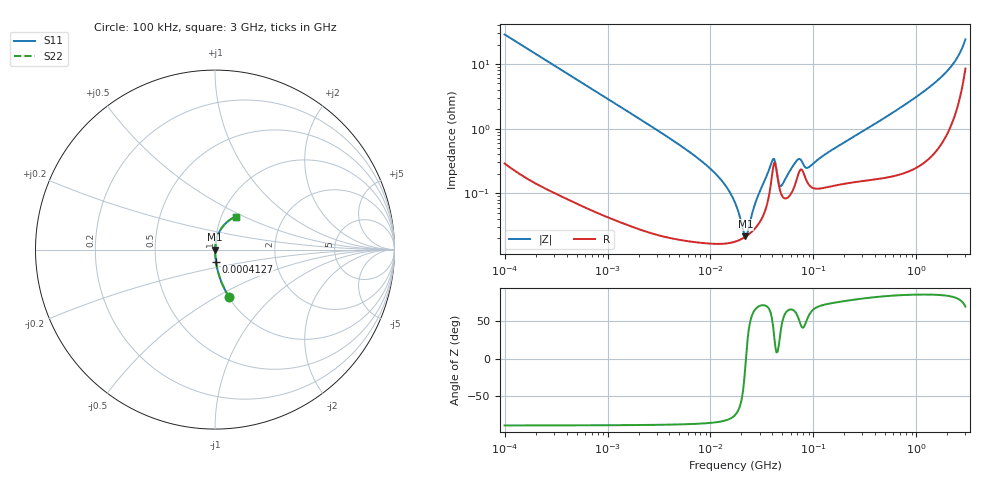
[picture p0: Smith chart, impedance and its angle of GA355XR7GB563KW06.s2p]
!Murata Part Number: GA355XR7GB563KW06
!These Parameters are Measured in Series Mode Connection
!Data Generated on Jun 19, 2026
!  o--ll--o
!Port1  Port2
!  o------o
!Operation Temp=25[degC], DC Bias Voltage=0[V]
!Freq. Start=100[kHz] Stop=3[GHz] 401[Steps]
# Hz S RI R 50
!Freq.(Hz) S11(Real) S11(Imag) S21(Real) S21(Imag) S12(Real) S12(Imag) S22(Real) S22(Imag)
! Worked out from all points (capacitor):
!   401 points, 100 kHz to 3 GHz, reference 50 ohm
!   read as one part in series: C = 55.4 nF near 105.3 kHz
!   lowest |Z| = 21.5 mohm at 21.84 MHz (marker M1)
!   series resonance near 22.14 MHz, so ESL is about 930 pH
!   S11 on the Smith chart (normalised r, x): 100 kHz: 1.01, -0.57; 412.7 kHz: 1.00, -0.14; 3 GHz: 1.17, +0.45
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100000  0.0782 -0.2636  0.9218 0.2636  0.9218 0.2636  0.0782 -0.2636
412671  0.00566 -0.0695  0.9943 0.0695  0.9943 0.0695  0.00566 -0.0695
562235  0.00327 -0.0512  0.9967 0.0512  0.9967 0.0512  0.00327 -0.0512
3161081  0.000305 -0.00908  0.9997 0.00908  0.9997 0.00908  0.000305 -0.00908
1.061445e7  0.00017 -0.00218  0.9998 0.00218  0.9998 0.00218  0.00017 -0.00218
1.446142e7  0.000169 -0.00121  0.9998 0.00121  0.9998 0.00121  0.000169 -0.00121
1.77727e7  0.000181 -0.000621  0.9998 0.000621  0.9998 0.000621  0.000181 -0.000621
2.184217e7  0.000212 -3.84e-05  0.9998 3.84e-05  0.9998 3.84e-05  0.000212 -3.84e-05
2.299754e7  0.000224 0.000111  0.9998 -0.000111  0.9998 -0.000111  0.000224 0.000111
2.826337e7  0.00031 0.000764  0.9997 -0.000764  0.9997 -0.000764  0.00031 0.000764
3.951212e7  0.0018 0.00249  0.9982 -0.00249  0.9982 -0.00249  0.0018 0.00249
4.160216e7  0.00294 0.00169  0.9971 -0.00169  0.9971 -0.00169  0.00294 0.00169
4.611977e7  0.00135 0.000427  0.9986 -0.000427  0.9986 -0.000427  0.00135 0.000427
4.855934e7  0.000983 0.000826  0.999 -0.000826  0.999 -0.000826  0.000983 0.000826
6.965816e7  0.00174 0.00276  0.9983 -0.00276  0.9983 -0.00276  0.00174 0.00276
7.525761e7  0.00234 0.00235  0.9977 -0.00235  0.9977 -0.00235  0.00234 0.00235
8.560801e7  0.00158 0.00189  0.9984 -0.00189  0.9984 -0.00189  0.00158 0.00189
9.738194e7  0.00122 0.0025  0.9988 -0.0025  0.9988 -0.0025  0.00122 0.0025
5.475153e8  0.00204 0.0162  0.998 -0.0162  0.998 -0.0162  0.00204 0.0162
1.746113e9  0.00951 0.0616  0.9905 -0.0616  0.9905 -0.0616  0.00951 0.0616
2.318426e9  0.0244 0.0995  0.9756 -0.0995  0.9756 -0.0995  0.0244 0.0995
3e9  0.1166 0.184  0.8834 -0.184  0.8834 -0.184  0.1166 0.184
